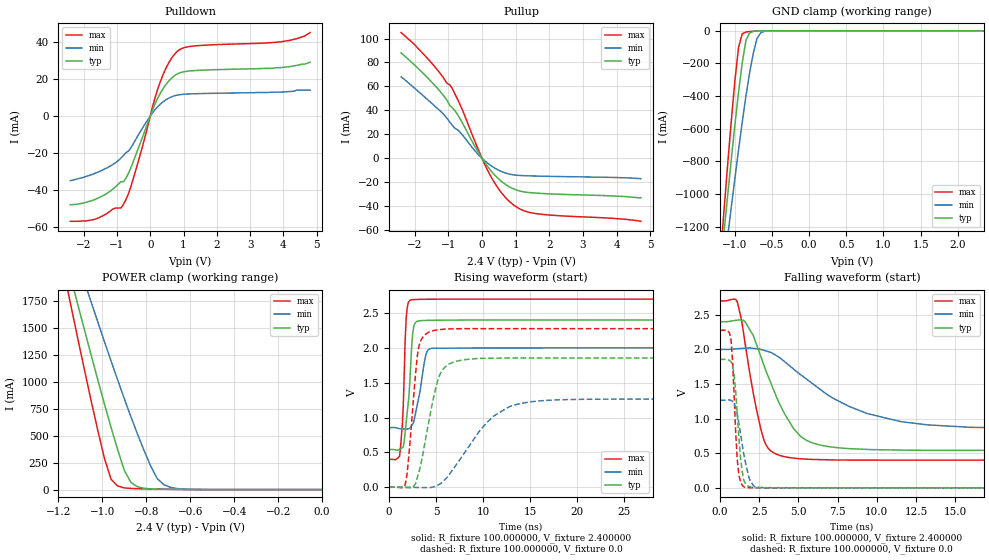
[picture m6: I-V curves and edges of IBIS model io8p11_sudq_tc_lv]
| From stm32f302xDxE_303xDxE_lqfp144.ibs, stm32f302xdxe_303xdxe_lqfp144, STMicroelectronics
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|   Model io8p11_sudq_tc_lv
[Model]  io8p11_sudq_tc_lv
Model_type I/O
Polarity   Non-Inverting
Enable   Active-Low
Vinl =   0.720000V
Vinh =   1.680000V
Vmeas =  1.200000V
Cref =   50.000000pF
Rref =   100.000000M
Vref =   0.0V
C_comp   1.378000pF   1.292700pF   1.486400pF
[Temperature Range]   25.000000   0.125000k   -40.000000
[Pullup Reference]   2.400000V   2.000000V   2.700000V
[Pulldown Reference]   0.0V   0.0V   0.0V
[POWER Clamp Reference]   2.400000V   2.000000V   2.700000V
[GND Clamp Reference]   0.0V   0.0V   0.0V
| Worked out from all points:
|   slope of the pulldown table from 0 to 0.36 V, typ, clamps not added: 25.7 ohm
|   slope of the pullup table from 0 to 0.36 V, typ, clamps not added: 26.8 ohm
|   GND clamp passes 1 mA (typ) near -0.67 V on its own axis
|   POWER clamp passes 1 mA (typ) near -0.60 V on its own axis
|   rising waveform, R_fixture 100.000000, V_fixture 2.400000: 20-80 % time 602ps typ, 876ps min, 369ps max; typ from 0.542 V to 2.4 V
|   rising waveform, R_fixture 100.000000, V_fixture 0.0: 20-80 % time 1.64ns typ, 4.29ns min, 857ps max; typ from 0 V to 1.85 V
|   falling waveform, R_fixture 100.000000, V_fixture 2.400000: 20-80 % time 2.14ns typ, 4.88ns min, 1.09ns max; typ from 2.4 V to 0.542 V
|   falling waveform, R_fixture 100.000000, V_fixture 0.0: 20-80 % time 379ps typ, 597ps min, 284ps max; typ from 1.85 V to 0 V
[Pulldown]
|Voltage   I(typ)   I(min)   I(max)
-2.4V     -47.8mA    -34.8mA    -56.7mA
-1.68V    -45.1mA    -31mA      -55.7mA
-1.12V    -39.3mA    -26.1mA    -50.05mA
-800mV    -35.33mA   -21.13mA   -47.42mA
-640mV    -30.33mA   -18.65mA   -41.16mA
-480mV    -23.12mA   -14mA      -31.94mA
240mV     10.22mA    5.339mA    15.38mA
480mV     17.22mA    8.864mA    26.1mA
800mV     22.59mA    11.27mA    34.68mA
1.36V     24.54mA    12.05mA    37.84mA
3.92V     26.1mA     12.9mA     40mA
4.8V      29mA       14mA       45mA
[Pullup]
|Voltage   I(typ)   I(min)   I(max)
-2.4V     88mA       68mA       105mA
-2V       77.9mA     58.5mA     95mA
-1.36V    59.6mA     42.5mA     75.1mA
-880mV    42.12mA    27.44mA    58.22mA
-560mV    28.45mA    18.75mA    39mA
-160mV    7.44mA     4.66mA     10.64mA
160mV     -6.607mA   -3.947mA   -9.704mA
480mV     -16.91mA   -9.806mA   -25.1mA
880mV     -24.9mA    -13.63mA   -37.75mA
1.2V      -27.87mA   -14.5mA    -43.37mA
1.6V      -29.13mA   -14.89mA   -46.24mA
4.72V     -33.1mA    -17.1mA    -52.7mA
[GND_clamp]
|Voltage   I(typ)   I(min)   I(max)
-2.4V     -7.358A    -6.372A    -8.78A
-1.2V     -1.489A    -1.65A     -1.416A
-1.15V    -1.254A    -1.461A    -1.124A
-1.1V     -1.024A    -1.273A    -838.2mA
-1.05V    -797.6mA   -1.088A    -563.1mA
-950mV    -374.6mA   -728.7mA   -100.8mA
-900mV    -194.3mA   -557.9mA   -18.01mA
-850mV    -56.94mA   -397.4mA   -7.08mA
-750mV    -3.582mA   -133.8mA   -2.771mA
-700mV    -1.516mA   -44.7mA    -1.516mA
-600mV    -235.4uA   -2.939mA   -209.5uA
2.35V     0A         0A         0A
[POWER_clamp]
|Voltage   I(typ)   I(min)   I(max)
-2.4V     9.979A     9.967A     9.901A
-1.17V    2.182A     2.481A     1.978A
-1.14V    1.945A     2.294A     1.683A
-1.11V    1.71A      2.108A     1.391A
-1.08V    1.476A     1.923A     1.102A
-1.05V    1.245A     1.739A     819.9mA
-960mV    578.2mA    1.196A     96.06mA
-900mV    179.5mA    846.7mA    16.04mA
-870mV    67.18mA    678.8mA    10.82mA
-780mV    6.749mA    219.9mA    5.853mA
-720mV    3.355mA    46.34mA    3.808mA
0V        0A         0A         0A
[Ramp]
| variable   typ   min   max
dV/dt_r  1.11318/1.63141n   0.75954/4.28204n   1.36572/0.85373n
dV/dt_f  1.11508/2.13656n   0.68690/4.87072n   1.37965/1.09067n
R_load = 100.000000
[Rising Waveform]
R_fixture= 100.000000
V_fixture= 2.400000
V_fixture_min= 2.000000
V_fixture_max= 2.700000
|time   V(typ)   V(min)   V(max)
0s        541.6mV    855mV      400.5mV
1.101ns   543.5mV    841.4mV    442.2mV
1.502ns   578.7mV    836.4mV    1.171V
1.802ns   920.8mV    836.3mV    2.412V
2.302ns   1.79V      865.3mV    2.689V
2.503ns   2.206V     908.3mV    2.692V
2.703ns   2.343V     996.5mV    2.694V
3.904ns   2.394V     1.905V     2.698V
4.505ns   2.396V     1.993V     2.699V
49.85ns   2.4V       2V         2.7V
[Rising Waveform]
R_fixture= 100.000000
V_fixture= 0.0
V_fixture_min= 0.0
V_fixture_max= 0.0
|time   V(typ)   V(min)   V(max)
0s        804.5pV    13.47nV    619.4pV
1.702ns   -3.054mV   -57.8uV    36.23mV
2.002ns   -5.707mV   -163.8uV   325.5mV
3.103ns   192.1mV    -3.615mV   1.982V
4.705ns   1.279V     5.489mV    2.248V
5.506ns   1.648V     56.64mV    2.264V
6.607ns   1.783V     224.2mV    2.273V
10.41ns   1.851V     931.3mV    2.276V
14.01ns   1.856V     1.204V     2.276V
49.85ns   1.855V     1.266V     2.276V
[Falling Waveform]
R_fixture= 100.000000
V_fixture= 2.400000
V_fixture_min= 2.000000
V_fixture_max= 2.700000
|time   V(typ)   V(min)   V(max)
0s        2.4V       2V         2.7V
1.101ns   2.422V     2.01V      2.688V
2.102ns   2.208V     2.016V     1.393V
2.803ns   1.77V      1.986V     689.5mV
4.104ns   1.075V     1.826V     450.8mV
5.105ns   752.6mV    1.641V     421.1mV
6.206ns   628.7mV    1.454V     408.9mV
9.409ns   554.6mV    1.072V     401.1mV
13.21ns   542.9mV    910.5mV    400.3mV
49.85ns   541.6mV    855mV      400.5mV
[Falling Waveform]
R_fixture= 100.000000
V_fixture= 0.0
V_fixture_min= 0.0
V_fixture_max= 0.0
|time   V(typ)   V(min)   V(max)
0s        1.855V     1.266V     2.276V
700.7ps   1.823V     1.264V     2.144V
800.8ps   1.77V      1.251V     1.84V
900.9ps   1.636V     1.209V     1.346V
1.101ns   1.072V     1.065V     407.5mV
1.301ns   450.2mV    796.9mV    94.19mV
1.602ns   69.57mV    387.6mV    7.759mV
2.102ns   7.654mV    43.94mV    1.545mV
2.803ns   1.773mV    4.216mV    818.8uV
49.85ns   804.5pV    13.47nV    619.4pV
